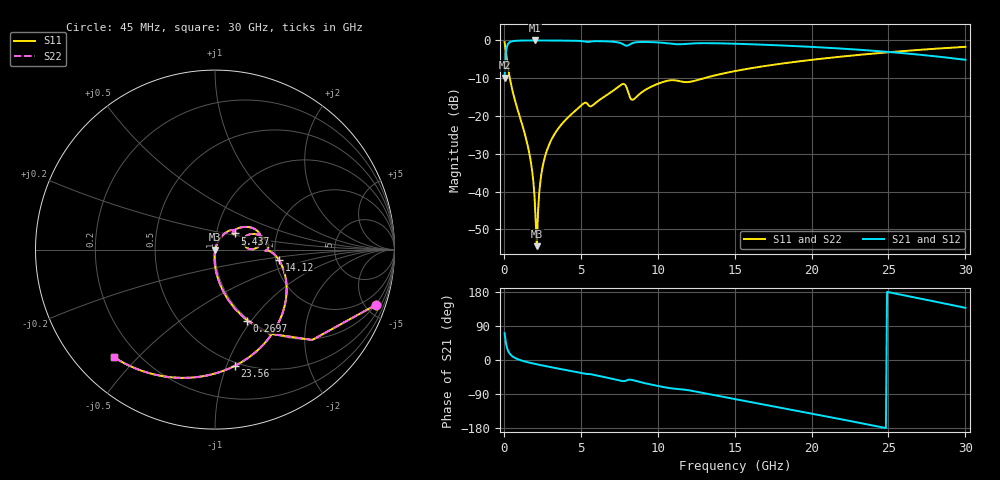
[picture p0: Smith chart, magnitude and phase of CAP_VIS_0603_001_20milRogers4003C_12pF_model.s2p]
! S-parameter model data by Modelithics Inc.  support@modelithics.com  813-866-6335  Tampa FL USA
! S-Parameter data specifications:
! Substrate: 20-mil Rogers 4003C, substrate thickness, H=0.508mm, Dielectric constant, Er=3.75
! PCB Mounting Pad Footprint: Pad width, PadW=0.90mm , Pad length, PadL=1.00mm , Pad gap, PadG (edge-to-edge)=1.00mm , Reference planes=3.0mm apart
! Created Wed Nov 18 13:26:20 2015
# hz S ma R 50
! 2 Port Network Data from SP1.SP block
! freq  magS11  angS11  magS21  angS21  magS12  angS12  magS22  angS22
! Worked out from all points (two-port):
!   401 points, 45 MHz to 30 GHz, reference 50 ohm
!   highest |S21| = -0.02 dB at 1.992 GHz (marker M1); lowest = -9.8 dB at 45 MHz (marker M2)
!   |S21| within 3 dB of the highest: 137.4 MHz to 24.89 GHz (24.76 GHz wide, 198 % of centre)
!   lowest |S11| = -54.4 dB at 2.142 GHz (marker M3), VSWR 1.00, Z = 50.2 + j0.0344 ohm
!   |S11| at or under -10 dB: 384.7 MHz to 13.01 GHz (12.63 GHz wide, 189 % of centre)
!   |S22| runs from -54.4 to -0.5 dB; largest |S21 - S12| = 0
!   S11 on the Smith chart (normalised r, x): 45 MHz: 0.98, -5.80; 269.7 MHz: 0.98, -0.95; 5.437 GHz: 1.23, +0.23; 14.12 GHz: 2.08, -0.27; 23.56 GHz: 0.47, -1.07; 30 GHz: 0.12, -0.43
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4.5e7  0.9465 -19.1  0.3225 70.9  0.3225 70.9  0.9465 -19.1
2.696625e8  0.4342 -65.6  0.9002 24.3  0.9002 24.3  0.4342 -65.6
5.692125e8  0.2108 -80.6  0.9766 9.1  0.9766 9.1  0.2108 -80.6
1.617638e9  0.03483 -94.1  0.9977 -6.6  0.9977 -6.6  0.03483 -94.1
1.8423e9  0.01831 -93.6  0.998 -8.7  0.998 -8.7  0.01831 -93.6
1.992075e9  0.008571 -88.7  0.9981 -10.1  0.9981 -10.1  0.008571 -88.7
2.14185e9  0.0019 10.4  0.9981 -11.4  0.9981 -11.4  0.0019 10.4
2.216738e9  0.005347 58.3  0.998 -12.1  0.998 -12.1  0.005347 58.3
2.516288e9  0.02128 70.2  0.9976 -14.6  0.9976 -14.6  0.02128 70.2
2.965612e9  0.04306 69.0  0.9967 -18.2  0.9967 -18.2  0.04306 69.0
3.714488e9  0.0762 64.0  0.9942 -24.1  0.9942 -24.1  0.0762 64.0
5.062462e9  0.1401 50.6  0.9789 -34.9  0.9789 -34.9  0.1401 50.6
5.4369e9  0.1443 38.7  0.9538 -36.9  0.9538 -36.9  0.1443 38.7
7.683525e9  0.2628 20.8  0.9039 -55.5  0.9039 -55.5  0.2628 20.8
8.357512e9  0.1637 13.2  0.9218 -52.9  0.9218 -52.9  0.1637 13.2
1.007992e10  0.2701 15.7  0.9378 -69.1  0.9378 -69.1  0.2701 15.7
1.412385e10  0.3601 -9.2  0.9135 -96.3  0.9135 -96.3  0.3601 -9.2
1.50225e10  0.3928 -15.3  0.9034 -103.2  0.9034 -103.2  0.3928 -15.3
2.003996e10  0.5543 -52.7  0.8198 -141.6  0.8198 -141.6  0.5543 -52.7
2.355968e10  0.6568 -80.3  0.7409 -169.4  0.7409 -169.4  0.6568 -80.3
2.505742e10  0.6982 -92.3  0.7022 178.5  0.7022 178.5  0.6982 -92.3
3e10  0.822 -133.0  0.5532 137.7  0.5532 137.7  0.822 -133.0
